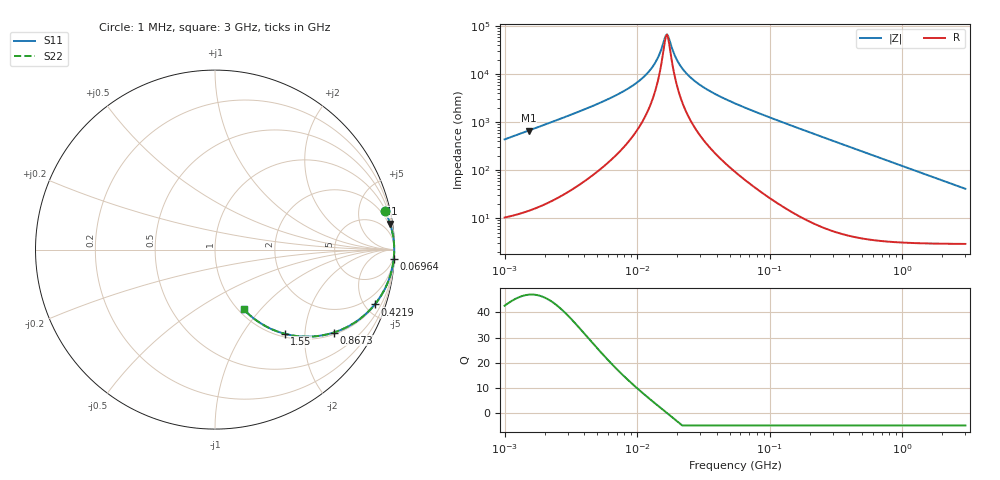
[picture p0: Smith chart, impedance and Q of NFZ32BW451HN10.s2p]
! NFZ32BW451HN10
# Hz S RI R 50
!Freq.(Hz) S11(Real) S11(Imag) S21(Real) S21(Imag) S12(Real) S12(Imag) S22(Real) S22(Imag)
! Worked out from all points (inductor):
!   401 points, 1 MHz to 3 GHz, reference 50 ohm
!   read as one part in series: L = 69.4 uH near 1.041 MHz
!   highest Q = 47.1 at 1.522 MHz (marker M1), where L = 69.9 uH
!   self-resonance near 16.48 MHz
!   S11 on the Smith chart (normalised r, x): 1 MHz: 1.21, +8.76; 69.64 MHz: 2, -37; 421.9 MHz: 1.08, -5.80; 867.3 MHz: 1.06, -2.82; 1.55 GHz: 1.06, -1.58; 3 GHz: 1.06, -0.82
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1000000  0.9459 0.2147  0.0541 -0.2147  0.0541 -0.2147  0.9459 0.2147
1522470  0.9752 0.1452  0.0248 -0.1452  0.0248 -0.1452  0.9752 0.1452
3823119  0.9951 0.0565  0.00495 -0.0565  0.00495 -0.0565  0.9951 0.0565
6696013  0.9976 0.0287  0.00238 -0.0287  0.00238 -0.0287  0.9976 0.0287
9600343  0.9982 0.016  0.00176 -0.016  0.00176 -0.016  0.9982 0.016
1.245355e7  0.9984 0.00823  0.00156 -0.00823  0.00156 -0.00823  0.9984 0.00823
1.461624e7  0.9985 0.00375  0.0015 -0.00375  0.0015 -0.00375  0.9985 0.00375
1.615473e7  0.9985 0.001  0.00148 -0.001  0.00148 -0.001  0.9985 0.001
1.681455e7  0.9985 -9.46e-05  0.00148 9.46e-05  0.00148 9.46e-05  0.9985 -9.46e-05
1.750132e7  0.9985 -0.00119  0.00148 0.00119  0.00148 0.00119  0.9985 -0.00119
1.896016e7  0.9985 -0.00339  0.00149 0.00339  0.00149 0.00339  0.9985 -0.00339
2.013356e7  0.9985 -0.00505  0.0015 0.00505  0.0015 0.00505  0.9985 -0.00505
2.459509e7  0.9984 -0.0107  0.00159 0.0107  0.00159 0.0107  0.9984 -0.0107
3.387922e7  0.9981 -0.0209  0.00192 0.0209  0.00192 0.0209  0.9981 -0.0209
5.477226e7  0.9968 -0.0404  0.00316 0.0404  0.00316 0.0404  0.9968 -0.0404
6.964249e7  0.9956 -0.0533  0.00441 0.0533  0.00441 0.0533  0.9956 -0.0533
2.094008e8  0.9697 -0.1646  0.0303 0.1646  0.0303 0.1646  0.9697 -0.1646
4.219165e8  0.8905 -0.3053  0.1095 0.3053  0.1095 0.3053  0.8905 -0.3053
8.005644e8  0.6964 -0.4494  0.3036 0.4494  0.3036 0.4494  0.6964 -0.4494
8.672962e8  0.6621 -0.4619  0.3379 0.4619  0.3379 0.4619  0.6621 -0.4619
1.54974e9  0.3881 -0.4689  0.6119 0.4689  0.6119 0.4689  0.3881 -0.4689
3e9  0.1599 -0.3327  0.8401 0.3327  0.8401 0.3327  0.1599 -0.3327
